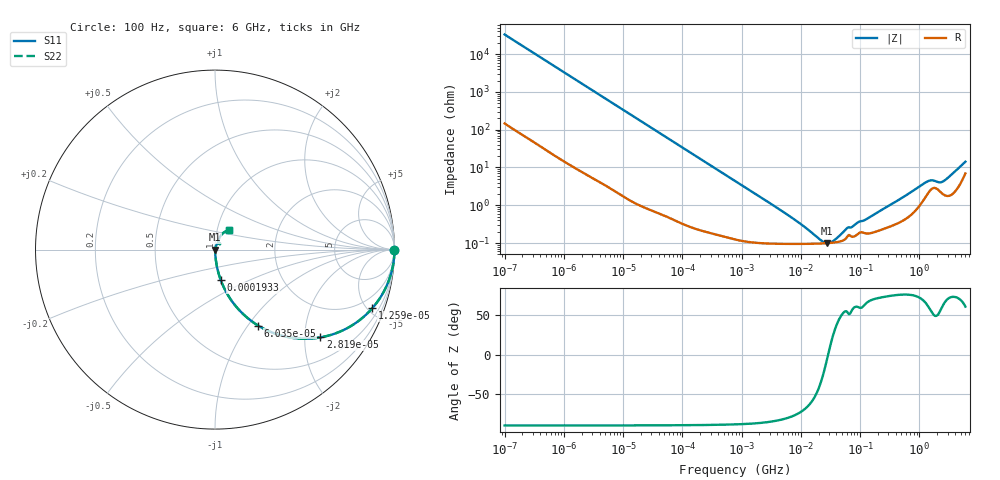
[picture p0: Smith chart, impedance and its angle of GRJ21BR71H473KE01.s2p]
!Murata Part Number: GRJ21BR71H473KE01
!These Parameters are Measured in Series Mode Connection
!Data Generated on Jun 19, 2026
!  o--ll--o
!Port1  Port2
!  o------o
!Operation Temp=25[degC], DC Bias Voltage=0[V]
!Freq. Start=100[Hz] Stop=6[GHz] 401[Steps]
# Hz S RI R 50
!Freq.(Hz) S11(Real) S11(Imag) S21(Real) S21(Imag) S12(Real) S12(Imag) S22(Real) S22(Imag)
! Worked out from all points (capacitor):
!   401 points, 100 Hz to 6 GHz, reference 50 ohm
!   read as one part in series: C = 47.9 nF near 109 Hz
!   lowest |Z| = 99.4 mohm at 27.84 MHz (marker M1)
!   series resonance near 28.9 MHz, so ESL is about 630 pH
!   S11 on the Smith chart (normalised r, x): 100 Hz: open; 12.59 kHz: 1.03, -5.34; 28.19 kHz: 1.02, -2.39; 60.35 kHz: 1.01, -1.12; 193.3 kHz: 1.00, -0.35; 6 GHz: 1.14, +0.25
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100  1 -0.00302  2.24e-05 0.00302  2.24e-05 0.00302  1 -0.00302
2008  0.9961 -0.0598  0.00387 0.0598  0.00387 0.0598  0.9961 -0.0598
5378  0.9742 -0.1561  0.0258 0.1561  0.0258 0.1561  0.9742 -0.1561
12592  0.8757 -0.3274  0.1243 0.3274  0.1243 0.3274  0.8757 -0.3274
28191  0.5876 -0.4891  0.4124 0.4891  0.4124 0.4891  0.5876 -0.4891
40335  0.4123 -0.4886  0.5877 0.4886  0.5877 0.4886  0.4123 -0.4886
60352  0.2406 -0.4233  0.7594 0.4233  0.7594 0.4233  0.2406 -0.4233
103284  0.0995 -0.2945  0.9005 0.2945  0.9005 0.2945  0.0995 -0.2945
193316  0.032 -0.1697  0.968 0.1697  0.968 0.1697  0.032 -0.1697
774597  0.00318 -0.044  0.9968 0.044  0.9968 0.044  0.00318 -0.044
6075234  0.000976 -0.0054  0.999 0.0054  0.999 0.0054  0.000976 -0.0054
1.555665e7  0.000957 -0.00157  0.999 0.00157  0.999 0.00157  0.000957 -0.00157
2.225763e7  0.000971 -0.00063  0.999 0.00063  0.999 0.00063  0.000971 -0.00063
2.784235e7  0.000989 -8.9e-05  0.999 8.9e-05  0.999 8.9e-05  0.000989 -8.9e-05
3.64232e7  0.00103 0.000562  0.999 -0.000562  0.999 -0.000562  0.00103 0.000562
5.960426e7  0.00141 0.00198  0.9986 -0.00198  0.9986 -0.00198  0.00141 0.00198
1.275994e8  0.0018 0.00386  0.9982 -0.00386  0.9982 -0.00386  0.0018 0.00386
3.124326e8  0.00277 0.00948  0.9972 -0.00948  0.9972 -0.00948  0.00277 0.00948
1.369159e9  0.0205 0.0363  0.9795 -0.0363  0.9795 -0.0363  0.0205 0.0363
2.240541e9  0.0235 0.0315  0.9765 -0.0315  0.9765 -0.0315  0.0235 0.0315
2.562649e9  0.0203 0.0374  0.9797 -0.0374  0.9797 -0.0374  0.0203 0.0374
6e9  0.0772 0.1072  0.9228 -0.1072  0.9228 -0.1072  0.0772 0.1072
